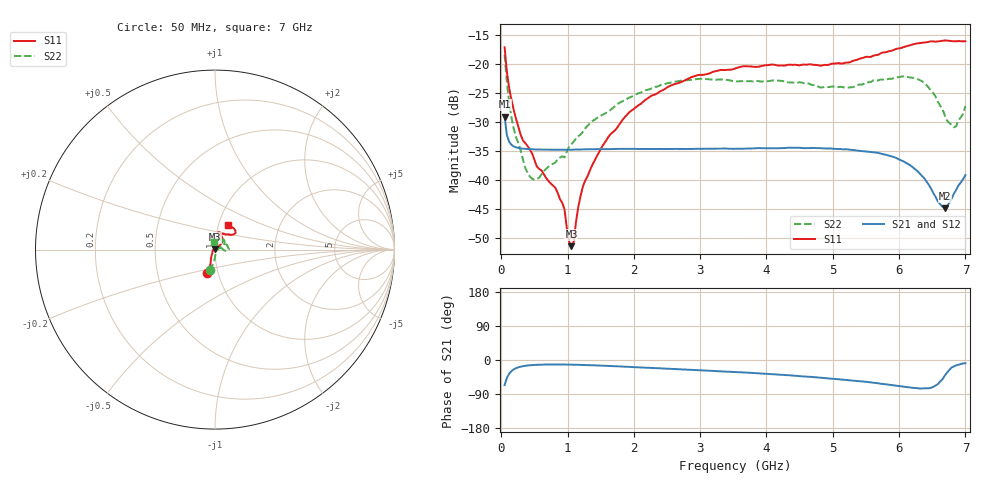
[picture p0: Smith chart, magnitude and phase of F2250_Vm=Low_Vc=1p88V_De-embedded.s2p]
! Integrated Device Technology
! Corporate Headquarters
! 6024 Silver Creek Valley Road
! San Jose, CA 95138  USA
! Phone:  1-408-284-8200
! Toll Free:  1-800-223-1366
! Webpage:  http://www.idt.com/
! Timing and RF Division
! 515 Groton Road, Suite 102
! Westford, MA 01886-6024
! Device:  F2250
! Description: Voltage Variable RF Attenuator
! Frequency:  50.0 -  6000.00 MHz
! Package:  3x3 mm Thin QFN Plastic Package: 16 pin
! Ports:  2 RF, 3 DC
!  Pin  1  = GND
!  Pin  2  = NC
!  Pin  3  = RF1  = Port 1
!  Pin  4  = NC
!  Pin  5  = GND
!  Pin  6  = GND
!  Pin  7  = GND
!  Pin  8  = GND
!  Pin  9  = NC
!  Pin 10  = RF2  = Port 2
!  Pin 11  = NC
!  Pin 12  = GND
!  Pin 13  = GND
!  Pin 14  = VCNTRL
!  Pin 15  = VDD
!  Pin 16  = VMODE
! Vcntrl:  1.880 Volts
! Vmode:  +0.000 Volts
! Vdd:  +3.30  Volts
! Current:  1.183 mA
! Data:  The device was measured on a the F2250 evaluation board which has
!  individual transmission lines to the RF pins.  Data was collected
!  using a calibrated network analyzer.  The evaluation board was
!  de-embedded using a TRL calibration technique.
!  The reference plane is the edge of the package pin.
! Misc:  SN 10
!  Action Tracker AT0258
! Date Measured:  2014-11-26
! Date:  2015-10-15  MJV
! Note:
!  Integrated Device Technology supplies this data as a sample of measured
!  data at the package pin for this product.  Your particular data for this
!  product may vary.
!  Data was taken at 25 degrees C.
!  Integrated Device Technology reserves the right to change this data at anytime.
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# GHz S dB R 50
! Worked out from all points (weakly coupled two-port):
!   201 points, 50 MHz to 7 GHz, reference 50 ohm
!   highest |S21| = -29.06 dB at 50 MHz (marker M1); lowest = -44.9 dB at 6.687 GHz (marker M2)
!   lowest |S11| = -51.3 dB at 1.058 GHz (marker M3), VSWR 1.01, Z = 49.9 + j0.233 ohm
!   |S11| at or under -10 dB: start of sweep to end of sweep
!   |S22| runs from -39.9 to -18.5 dB; largest |S21 - S12| = 5.9e-05
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0.05  -17.17 -108.5  -29.06 -66.2  -29.06 -66.2  -18.46 -104.5
0.08475  -21.44 -107.2  -32.28 -47.2  -32.28 -47.2  -23.27 -94.1
0.189  -28.01 -119.4  -34.20 -24.6  -34.20 -24.6  -31.23 -83.6
0.328  -33.20 -133.3  -34.59 -16.2  -34.58 -16.2  -36.52 -55.5
0.43225  -34.78 -144.1  -34.68 -13.8  -34.68 -13.8  -39.39 -28.0
0.57125  -38.06 -159.9  -34.74 -12.4  -34.74 -12.4  -39.57 -8.1
0.91875  -43.88 158.1  -34.78 -11.9  -34.78 -11.9  -35.90 11.9
0.9535  -45.00 170.3  -34.78 -12.0  -34.78 -12.0  -36.07 16.6
1.023  -50.56 143.1  -34.77 -12.1  -34.76 -12.1  -34.27 18.4
1.05775  -51.33 120.7  -34.77 -12.2  -34.77 -12.2  -33.82 19.8
1.0925  -50.58 86.3  -34.76 -12.3  -34.75 -12.3  -33.37 19.0
1.162  -44.55 54.2  -34.74 -12.6  -34.74 -12.6  -32.44 17.0
1.2315  -41.05 42.9  -34.72 -12.9  -34.72 -12.9  -31.65 16.4
1.6485  -32.09 41.4  -34.66 -15.8  -34.65 -15.8  -27.92 25.2
2.37825  -24.87 47.1  -34.63 -21.8  -34.63 -21.9  -23.79 33.9
3.525  -20.82 72.4  -34.61 -31.8  -34.60 -31.8  -23.01 60.8
4.7065  -20.18 72.3  -34.46 -45.1  -34.46 -45.1  -23.67 63.8
5.85325  -17.83 40.4  -35.81 -65.4  -35.81 -65.5  -22.57 9.2
6.33975  -16.41 40.9  -39.22 -75.1  -39.22 -75.1  -22.95 -4.8
6.68725  -16.00 48.8  -44.86 -41.7  -44.86 -41.4  -28.81 14.6
6.82625  -16.14 53.5  -42.33 -17.0  -42.30 -16.9  -30.91 51.2
7  -16.13 63.2  -39.11 -8.5  -39.07 -8.6  -27.27 94.2
